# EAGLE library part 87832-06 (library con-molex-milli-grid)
HEADER
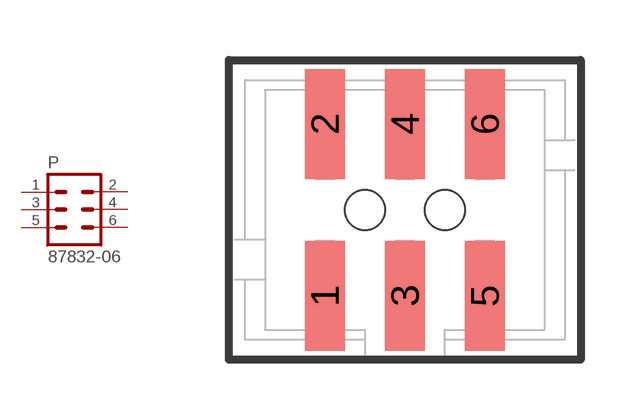
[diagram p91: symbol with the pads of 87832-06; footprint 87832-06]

Designator prefix P

## 87832-06  [87832-06]
1  1  pas
2  2  pas
3  3  pas
4  4  pas
5  5  pas
6  6  pas

## Footprint 87832-06 (pad centres in mm)
HEADER SMD Dual Row, Shrouded, Vertical
smd 1 x 2.75: 1 -2,-2.15; 2 -2,2.15; 3 0,-2.15; 4 0,2.15; 5 2,-2.15; 6 2,2.15
hole 1 at -1,0
hole 1 at 1,0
